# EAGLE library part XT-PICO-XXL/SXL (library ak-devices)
AK-NORD XT-PICO-XXL/SXL
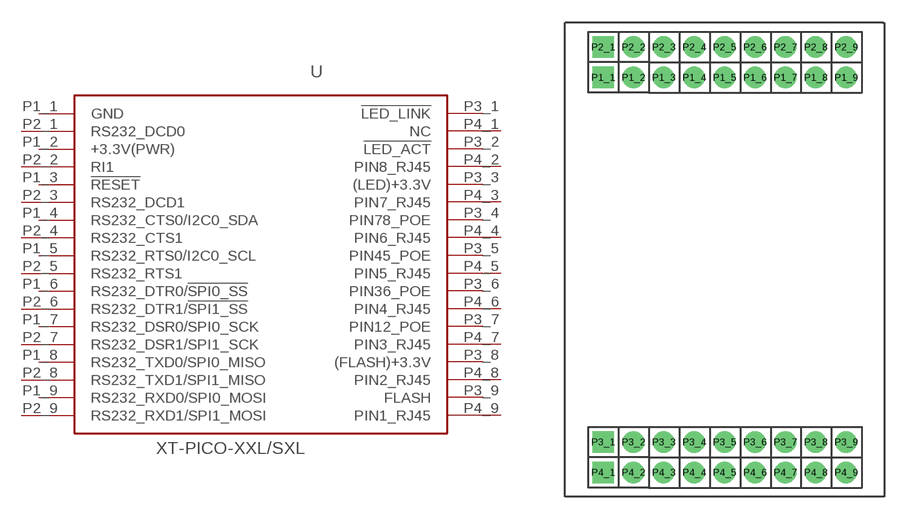
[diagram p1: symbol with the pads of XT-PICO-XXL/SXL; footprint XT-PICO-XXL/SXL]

Designator prefix -

## XT-PICO-XXL/SXL  [XT-PICO-XXL/SXL]
P1_1  GND  pwr
P1_2  +3.3V(PWR)  pwr
P1_3  !RESET  pas
P1_4  RS232_CTS0/I2C0_SDA  pas
P1_5  RS232_RTS0/I2C0_SCL  pas
P1_6  RS232_DTR0/!SPI0_SS!  pas
P1_7  RS232_DSR0/SPI0_SCK  pas
P1_8  RS232_TXD0/SPI0_MISO  pas
P1_9  RS232_RXD0/SPI0_MOSI  pas
P2_1  RS232_DCD0  pas
P2_2  RI1  pas
P2_3  RS232_DCD1  pas
P2_4  RS232_CTS1  pas
P2_5  RS232_RTS1  pas
P2_6  RS232_DTR1/!SPI1_SS!  pas
P2_7  RS232_DSR1/SPI1_SCK  pas
P2_8  RS232_TXD1/SPI1_MISO  pas
P2_9  RS232_RXD1/SPI1_MOSI  pas
P3_1  !LED_LINK  pas
P3_2  !LED_ACT  pas
P3_3  (LED)+3.3V  pas
P3_4  PIN78_POE
P3_5  PIN45_POE
P3_6  PIN36_POE
P3_7  PIN12_POE
P3_8  (FLASH)+3.3V  pas
P3_9  FLASH  pas
P4_1  NC  nc
P4_2  PIN8_RJ45
P4_3  PIN7_RJ45
P4_4  PIN6_RJ45
P4_5  PIN5_RJ45
P4_6  PIN4_RJ45
P4_7  PIN3_RJ45
P4_8  PIN2_RJ45
P4_9  PIN1_RJ45

## Footprint XT-PICO-XXL/SXL (pad centres in mm)
AK-NORD XT-PICO-XXL/SXL
drill 0.813 pad 1.422 square: P1_1 -8,12; P2_1 -8,14; P3_1 -8,-12; P4_1 -8,-14
drill 0.813 pad 1.422: P1_2 -6,12; P1_3 -4,12; P1_4 -2,12; P1_5 0,12; P1_6 2,12; P1_7 4,12; P1_8 6,12; P1_9 8,12; P2_2 -6,14; P2_3 -4,14; P2_4 -2,14; P2_5 0,14; P2_6 2,14; P2_7 4,14; P2_8 6,14; P2_9 8,14; P3_2 -6,-12; P3_3 -4,-12; P3_4 -2,-12; P3_5 0,-12; P3_6 2,-12; P3_7 4,-12; P3_8 6,-12; P3_9 8,-12; P4_2 -6,-14; P4_3 -4,-14; P4_4 -2,-14; P4_5 0,-14; P4_6 2,-14; P4_7 4,-14; P4_8 6,-14; P4_9 8,-14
